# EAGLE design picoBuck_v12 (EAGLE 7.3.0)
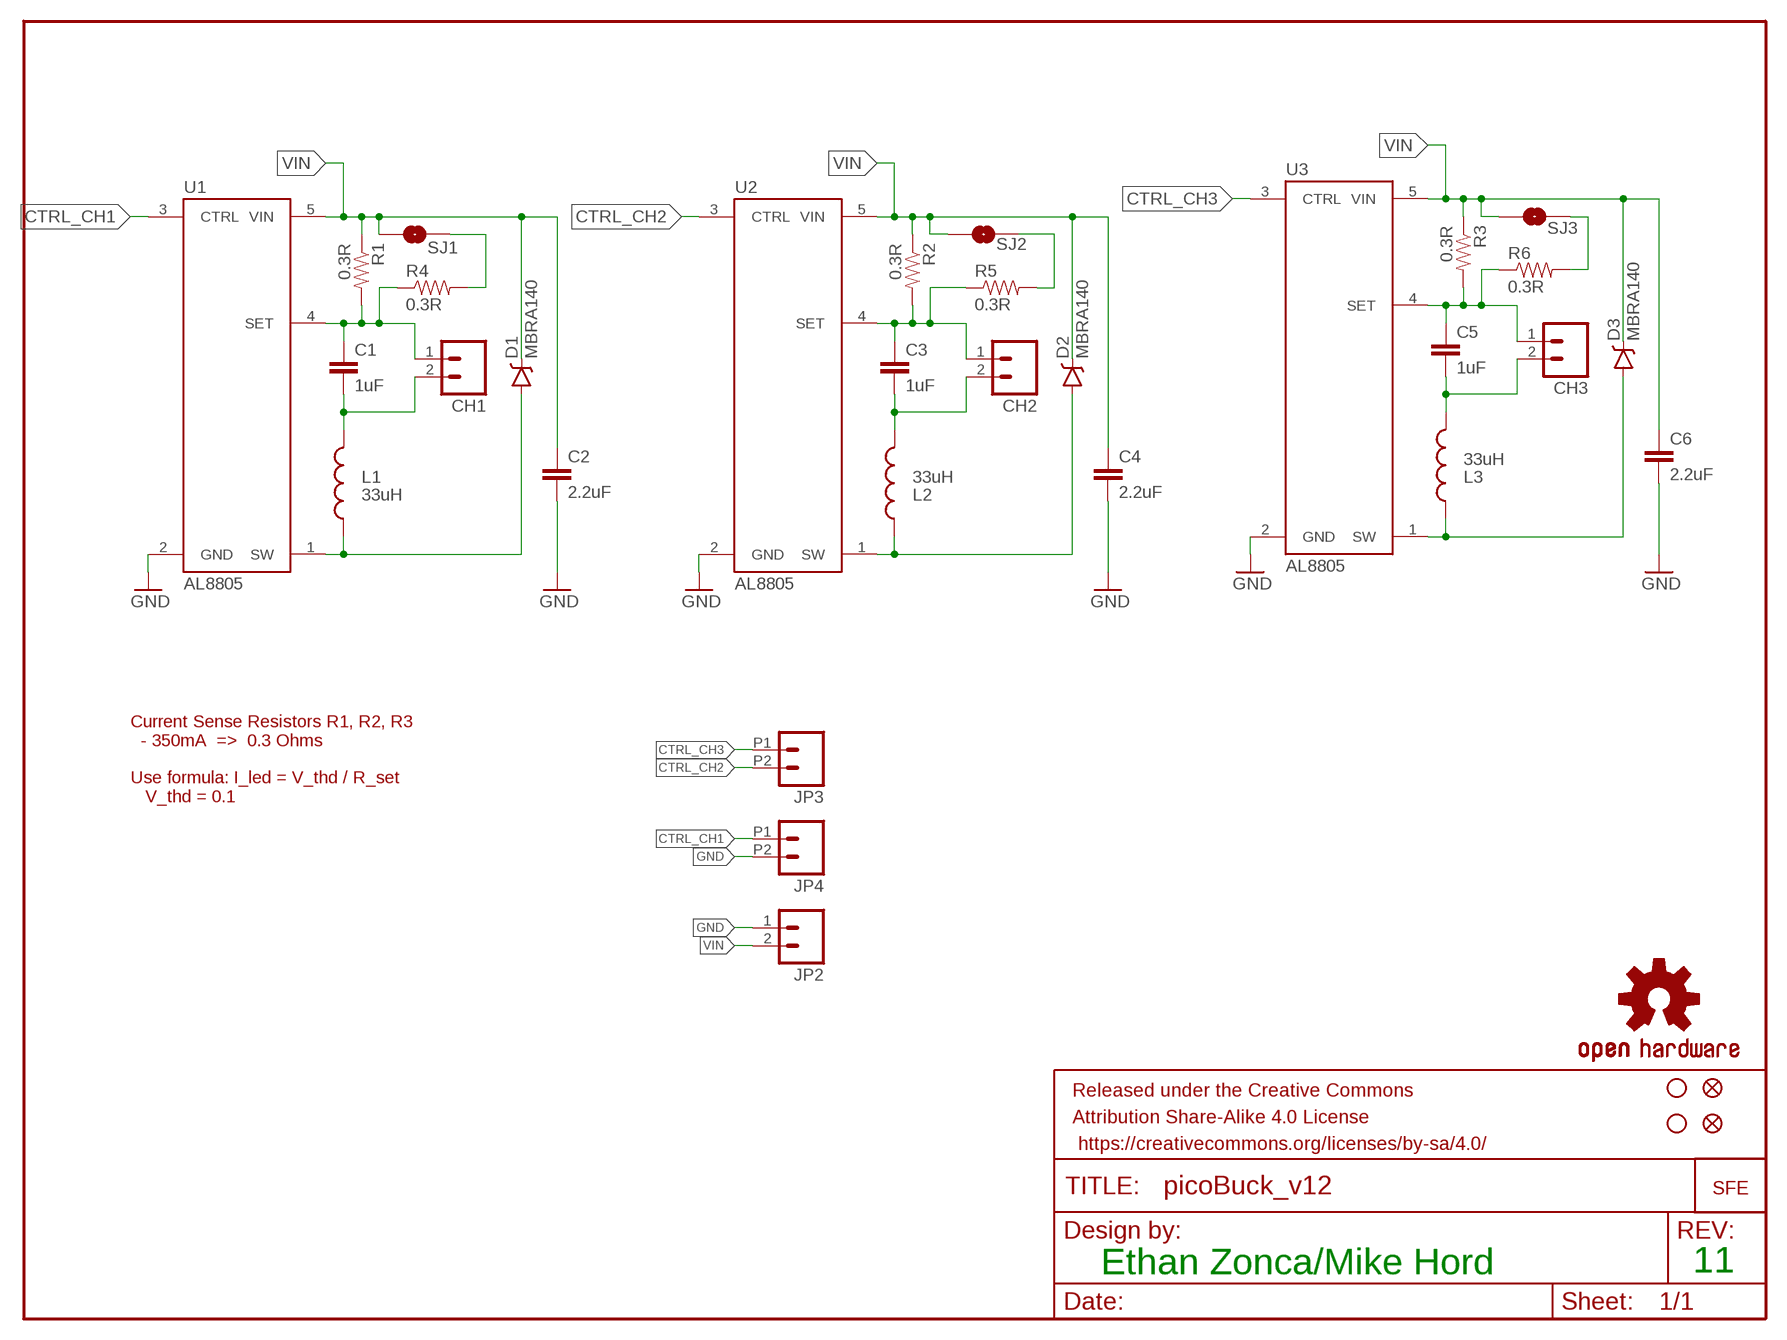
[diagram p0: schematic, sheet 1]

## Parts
C1  1uF  1.0UF-25V-+80/-20(0805)  [0805]
C2  2.2uF  2.2UF-25V-+80/-20(0805)  [0805]
C3  1uF  1.0UF-25V-+80/-20(0805)  [0805]
C4  2.2uF  2.2UF-25V-+80/-20(0805)  [0805]
C5  1uF  1.0UF-25V-+80/-20(0805)  [0805]
C6  2.2uF  2.2UF-25V-+80/-20(0805)  [0805]
CH1  M023.5MM_LOCK  [SCREWTERMINAL-3.5MM-2_LOCK]
CH2  M023.5MM_LOCK  [SCREWTERMINAL-3.5MM-2_LOCK]
CH3  M023.5MM_LOCK  [SCREWTERMINAL-3.5MM-2_LOCK]
D1  MBRA140  DIODE-SCHOTTKY-MBRA140  [SMA-DIODE]
D2  MBRA140  DIODE-SCHOTTKY-MBRA140  [SMA-DIODE]
D3  MBRA140  DIODE-SCHOTTKY-MBRA140  [SMA-DIODE]
FID1  FIDUCIALUFIDUCIAL  [MICRO-FIDUCIAL]
FID2  FIDUCIALUFIDUCIAL  [MICRO-FIDUCIAL]
FRAME1  FRAME-LETTER  [CREATIVE_COMMONS]
JP2  M023.5MM_LOCK  [SCREWTERMINAL-3.5MM-2_LOCK]
JP3  M022.54MM_SCREWTERM  [1X02_2.54_SCREWTERM]
JP4  M022.54MM_SCREWTERM  [1X02_2.54_SCREWTERM]
L1  33uH  INDUCTORBOURNS_SRN6045  [SRN6045]
L2  33uH  INDUCTORBOURNS_SRN6045  [SRN6045]
L3  33uH  INDUCTORBOURNS_SRN6045  [SRN6045]
LOGO1  OSHW-LOGOS  [OSHW-LOGO-S]
LOGO2  LOGO-SFENEW  [SFE-NEW-WEBLOGO]
R1  0.3R  0.3OHM-1/8W-1%(0805)  [0805]
R2  0.3R  0.3OHM-1/8W-1%(0805)  [0805]
R3  0.3R  0.3OHM-1/8W-1%(0805)  [0805]
R4  0.3R  0.3OHM-1/8W-1%(0805)  [0805]
R5  0.3R  0.3OHM-1/8W-1%(0805)  [0805]
R6  0.3R  0.3OHM-1/8W-1%(0805)  [0805]
SJ1  JUMPER-PAD-2-NO  [PAD-JUMPER-2-NO_NO_SILK]
SJ2  JUMPER-PAD-2-NO  [PAD-JUMPER-2-NO_NO_SILK]
SJ3  JUMPER-PAD-2-NO  [PAD-JUMPER-2-NO_NO_SILK]
STANDOFF1  STAND-OFF  [STAND-OFF]
STANDOFF2  STAND-OFF  [STAND-OFF]
U1  AL8805  [SOT23-5]
U2  AL8805  [SOT23-5]
U3  AL8805  [SOT23-5]

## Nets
CTRL_CH1: JP4.P1 U1.3(CTRL)
CTRL_CH2: JP3.P2 U2.3(CTRL)
CTRL_CH3: JP3.P1 U3.3(CTRL)
GND: C2.2 C4.2 C6.2 JP2.1 JP4.P2 U1.2(GND) U2.2(GND) U3.2(GND)
IND1-1: D1.A L1.1 U1.1(SW)
IND2-1: D2.A L2.1 U2.1(SW)
IND3-1: D3.A L3.1 U3.1(SW)
N$1: C5.1 CH3.1 R3.2 R6.1 U3.4(SET)
N$2: R4.2 SJ1.2
N$3: R5.2 SJ2.2
N$5 [power]: C1.2 CH1.2 L1.2
N$7: R6.2 SJ3.2
N$9 [power]: C3.2 CH2.2 L2.2
N$11: C1.1 CH1.1 R1.2 R4.1 U1.4(SET)
N$13: C3.1 CH2.1 R2.2 R5.1 U2.4(SET)
N$16 [power]: C5.2 CH3.2 L3.2
VIN: C2.1 C4.1 C6.1 D1.C D2.C D3.C JP2.2 R1.1 R2.1 R3.1 SJ1.1 SJ2.1 SJ3.1 U1.5(VIN) U2.5(VIN) U3.5(VIN)

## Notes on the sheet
- Current Sense Resistors R1, R2, R3
    - 350mA  =>  0.3 Ohms
  
  Use formula: I_led = V_thd / R_set
     V_thd = 0.1
- Ethan Zonca/Mike Hord | 11

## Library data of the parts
C1 C3 C5 = SparkFun-Capacitors:1.0UF-25V-+80/-20(0805); PROD_ID: CAP-11625; VALUE: 1.0uF
C2 C4 C6 = SparkFun-Capacitors:2.2UF-25V-+80/-20(0805); PROD_ID: CAP-11624
CH1-CH3 JP2 = SparkFun:M02: Header 2
D1-D3 = SparkFun-DiscreteSemi:DIODE-SCHOTTKY: Schottky diodes in SFE's production catalog; PROD_ID: DIO-08053
FID1 FID2 = SparkFun-Aesthetics:FIDUCIAL: Fiducial Alignment Points
FRAME1 = SparkFun-Aesthetics:FRAME-LETTER: Schematic Frame
JP3 JP4 = SparkFun-Connectors:M02: Standard 2-pin 0.1" header. Use with
L1-L3 = SparkFun-Passives:INDUCTOR: Inductors; PROD_ID: NDUC-11627
LOGO1 = SparkFun-Aesthetics:OSHW-LOGO: Open Source Hardware Logo This logo indicates the piece of hardware it is found on incorporates a OSHW license and/or adheres to the definition of open source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
LOGO2 = SparkFun-Aesthetics:LOGO-SFE: Spark Fun Electronics PCB Logo
R1-R6 = SparkFun-Resistors:0.3OHM-1/8W-1%(0805); PROD_ID: RES-11622; VALUE: 0.3
SJ1-SJ3 = SparkFun-Passives:JUMPER-PAD-2-NO
STANDOFF1 STANDOFF2 = SparkFun-Electromechanical:STAND-OFF: #4 Stand Off
U1-U3 = SparkFun-PowerIC:AL8805: Constant current LED driver PWM-able 1MHz switch freq 6V-36V Up to 1A LED current; PROD_ID: IC-11626; VALUE: AL8805WS

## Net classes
0 default: width 0.254 mm
1 power: width 0.508 mm

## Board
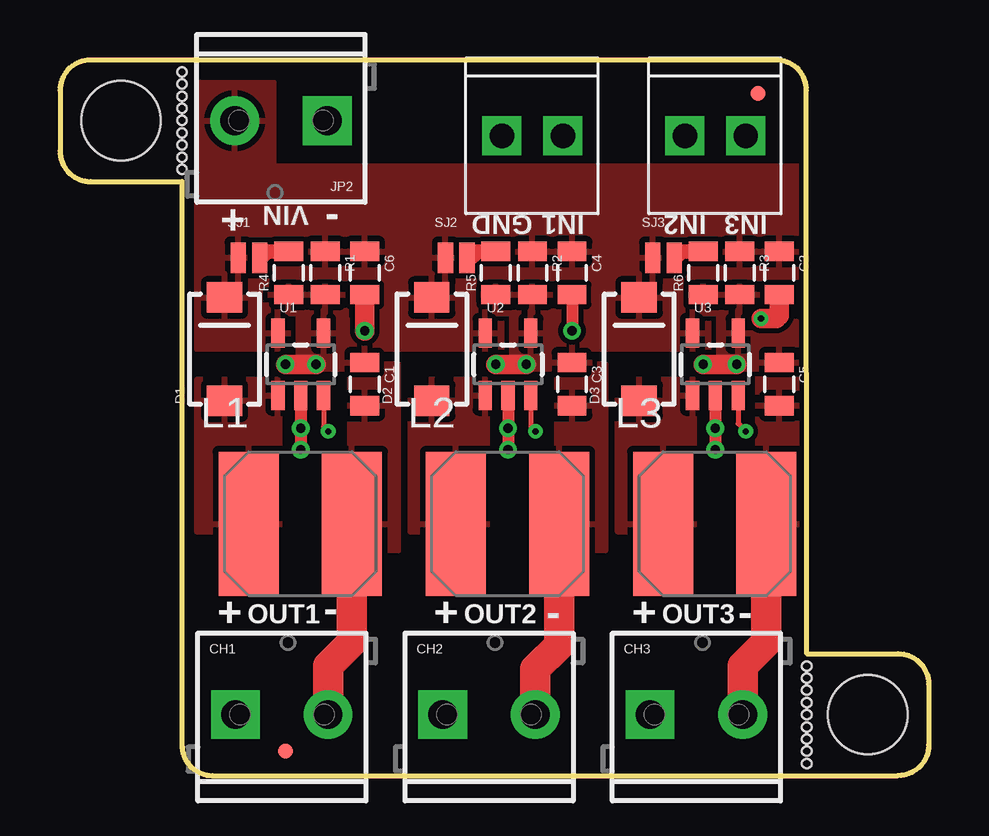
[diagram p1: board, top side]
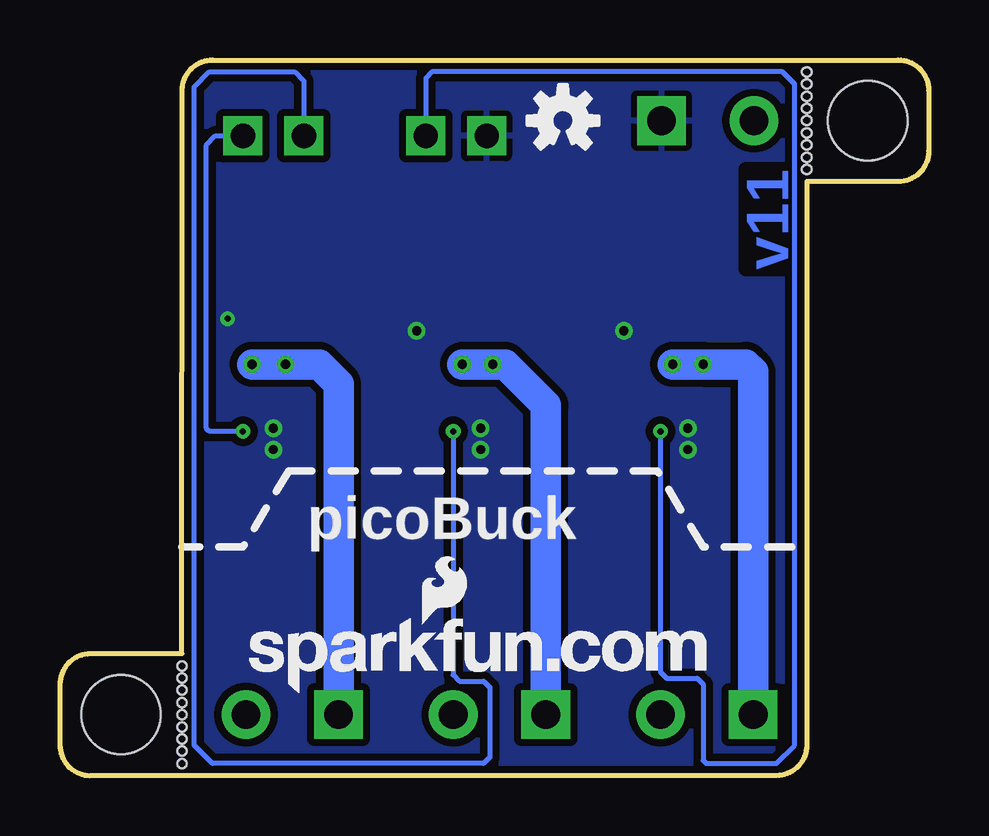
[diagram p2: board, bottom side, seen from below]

Size 36.2 x 29.84 mm. Coordinates in mm from the lower left corner, seen from the top.
Outline: 34.91,0 6.35,0 arc-90 5.08,1.27 5.08,24.77 1.27,24.77 arc-90 0,26.04 0,28.57 arc-90 1.27,29.84 29.83,29.84 arc-90 31.1,28.57 31.12,5.08 34.92,5.08 arc-90 36.2,3.81 36.2,1.27 arc-90 34.92,0
Copper layers (1*16): Top 0.035mm / dielectric 1.5mm / Bottom 0.035mm
Design rules "SparkFun-2-layer": minimum track width 7mil, minimum drill 15mil, track to track 8mil, track to pad 8mil, pad to pad 8mil, via to via 8mil, smd to smd 8mil, copper to edge 8mil, drill to drill 8mil, minimum pad ring 12mil, minimum via ring 7mil, stop-mask expansion 4mil, vias tented up to drill 20mil, thermal gap 10mil
Holes 0.38 mm at 31.12,4.57 31.12,4.06 31.12,3.56 31.12,3.05 31.12,2.54 31.12,2.03 31.12,1.52 31.12,1.02 31.12,0.51 5.08,29.34 5.08,28.83 5.08,28.32 5.08,27.81 5.08,27.3 5.08,26.8 5.08,26.29 5.08,25.78 5.08,25.27

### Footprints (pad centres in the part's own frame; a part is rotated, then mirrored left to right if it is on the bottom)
0805 = smd 0.8 x 1.2: 1 -0.9,0; 2 0.9,0
SCREWTERMINAL-3.5MM-2_LOCK = drill 1.2 pad 2.032 square: 1 -0.178,0 | drill 1.2 pad 2.032: 2 3.678,0
SMA-DIODE = smd 1.27 x 1.47: A -2.15,0; C 2.15,0
MICRO-FIDUCIAL = smd 0.635 x 0.635: 1 0,0
1X02_2.54_SCREWTERM = drill 1.016 square: P1 2.54,0; P2 0,0
SRN6045 = smd 2.5 x 6: 1 -2.175,-0.175; 2 2.125,-0.175
PAD-JUMPER-2-NO_NO_SILK = smd 0.635 x 1.27: 1 -0.45,0; 2 0.45,0
STAND-OFF = hole 3.302: 0,0
SOT23-5 = smd 0.55 x 1.2: 1 -0.95,-1.3; 2 0,-1.3; 3 0.95,-1.3; 4 0.95,1.3; 5 -0.95,1.3

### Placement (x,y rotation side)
C1  12.7,16.32 270 top
C2  29.97,20.95 270 top
C3  21.34,16.32 270 top
C4  21.34,20.95 270 top
C5  29.97,16.32 270 top
C6  12.7,20.95 270 top
CH1  7.49,2.54 0 top
CH2  16.13,2.54 0 top
CH3  24.77,2.54 0 top
D1  6.86,17.78 90 top
D2  15.49,17.78 90 top
D3  24.13,17.78 90 top
FID1  9.4,1.02 0 top
FID2  29.08,28.45 0 top
FRAME1  not placed on the board
JP2  10.95,27.3 180 top
JP3  26.03,26.67 0 top
JP4  18.41,26.67 0 top
L1  10.03,10.67 0 top
L2  18.67,10.67 0 top
L3  27.3,10.67 0 top
LOGO1  15.24,27.3 0 bottom
LOGO2  28.32,3.43 0 bottom
R1  11.05,20.95 270 top
R2  19.69,20.95 270 top
R3  28.32,20.95 270 top
R4  9.53,20.95 90 top
R5  18.16,20.95 90 top
R6  26.8,20.95 90 top
SJ1  7.87,21.59 0 top
SJ2  16.51,21.59 0 top
SJ3  25.15,21.59 0 top
STANDOFF1  2.54,27.3 0 top
STANDOFF2  33.66,2.54 0 top
U1  10.03,17.14 0 top
U2  18.67,17.14 0 top
U3  27.3,17.14 0 top

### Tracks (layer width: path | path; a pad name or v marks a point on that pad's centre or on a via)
CTRL_CH1  (via drill 0.25)
  Top 0.203: U1.3 10.98,14.54 v11.18,14.35
  Bottom 0.203: v11.18,14.35 11.18,4.32 10.92,4.06 9.65,4.06 9.4,3.81 9.4,0.64 9.27,0.51 6.35,0.51 5.59,1.27 5.59,28.83 6.1,29.34 20.7,29.34 20.95,29.08 JP4.P1
CTRL_CH2  (via drill 0.25)
  Top 0.203: U2.3 19.62,14.54 v19.81,14.35
  Bottom 0.203: v19.81,14.35 19.81,4.19 19.56,3.94 18.54,3.94 18.29,3.68 18.29,0.76 18.54,0.51 29.84,0.51 30.61,1.27 30.61,28.7 29.97,29.34 26.42,29.34 26.03,28.96 JP3.P2
CTRL_CH3  (via drill 0.25)
  Top 0.203: U3.3 28.26,14.67 v28.58,14.35
  Bottom 0.203: v28.58,14.35 29.97,14.35 30.1,14.48 30.1,26.29 29.72,26.67 JP3.P1
GND  (via drill 0.25, 0.38)
  Top 0.508: U1.2 v10.03,14.48 v10.03,13.59 | U2.2 v18.67,14.48 v18.67,13.59 | U3.2 v27.3,14.48 v27.3,13.59 | C4.2 v21.34,18.54
  Top 0.813: C6.2 v12.7,18.54 | C2.2 29.97,19.18 29.84,19.05 v29.21,19.05
  pour Bottom (isolate 0.305): 5.11,29.82 31.12,29.84 31.12,0 5.08,0
IND1-1
  pour Top (isolate 0.203, rank 3): 5.71,16.51 9.14,16.51 9.14,10.16 5.71,10.16
IND2-1
  pour Top (isolate 0.203): 14.61,16.51 17.78,16.51 17.78,10.16 14.61,10.16
IND3-1
  pour Top (isolate 0.203): 23.24,16.51 26.42,16.51 26.42,10.16 23.24,10.16
N$1  (via drill 0.38)
  Top 0.813: v26.8,17.14 v28.19,17.14
  Bottom 1.27: CH3.1 24.59,16.33 25.4,17.14 v26.8,17.14 v28.19,17.14
  pour Top (isolate 0.203): 27.43,16.95 30.73,16.95 30.73,18.92 29.59,18.92 29.46,19.05 29.46,20.38 26.26,20.38 26.26,19.27 27.43,19.27
N$2
  Top 0.61: 8.64,21.84 8.38,21.59 SJ1.2 8.59,21.86 R4.2
N$3
  Top 0.61: 17.27,21.72 17.14,21.59 SJ2.2 17.23,21.86 R5.2
N$5
  Top 1.27: CH1.2 11.17,4.57 12.16,5.55 L1.2
  pour Top (isolate 0.203, rank 3): 12.07,17.14 12.07,9.4 14.1,9.4 14.1,17.14
N$7
  Top 0.61: 25.91,21.84 25.65,21.59 SJ3.2 25.86,21.86 R6.2
N$9
  Top 1.27: L2.2 20.79,5.43 19.81,4.44 CH2.2
  pour Top (isolate 0.203, rank 3): 20.7,17.14 20.7,9.4 22.73,9.4 22.73,17.14
N$11  (via drill 0.38)
  Top 0.813: v10.67,17.14 v9.4,17.14
  Bottom 1.27: CH1.1 7.31,16.84 7.62,17.14 v9.4,17.14 v10.67,17.14
  pour Top (isolate 0.203): 9.91,16.95 13.21,16.95 13.21,18.92 12.07,18.92 11.94,19.05 11.94,20.38 8.73,20.38 8.73,19.27 9.91,19.27
N$13  (via drill 0.38)
  Top 0.813: v18.16,17.14 v19.43,17.14
  Bottom 1.27: CH2.1 15.95,15.44 17.65,17.14 v18.16,17.14 v19.43,17.14
  pour Top (isolate 0.203): 18.8,16.95 22.1,16.95 22.1,18.92 20.95,18.92 20.83,19.05 20.83,20.38 17.62,20.38 17.62,19.27 18.8,19.27
N$16
  Top 1.27: CH3.2 28.44,4.57 29.43,5.55 L3.2
  pour Top (isolate 0.203, rank 3): 29.08,17.14 29.08,9.4 31.12,9.4 31.12,17.14
VIN
  pour Top (isolate 0.203, rank 2): 5.71,28.89 8.89,28.89 8.89,25.4 31.12,25.4 31.12,17.78 5.71,17.78

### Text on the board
Bottom: v11
tPlace: + | VIN | - | GND | IN1 | IN2 | IN3 | + | OUT1 | - | + | OUT2 | - | + | OUT3 | -
bPlace: picoBuck
Measures: #4-40 typ. | (typ.) | (typ.) | Units are inches
tDocu: Ethan Zonca/Mike Hord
